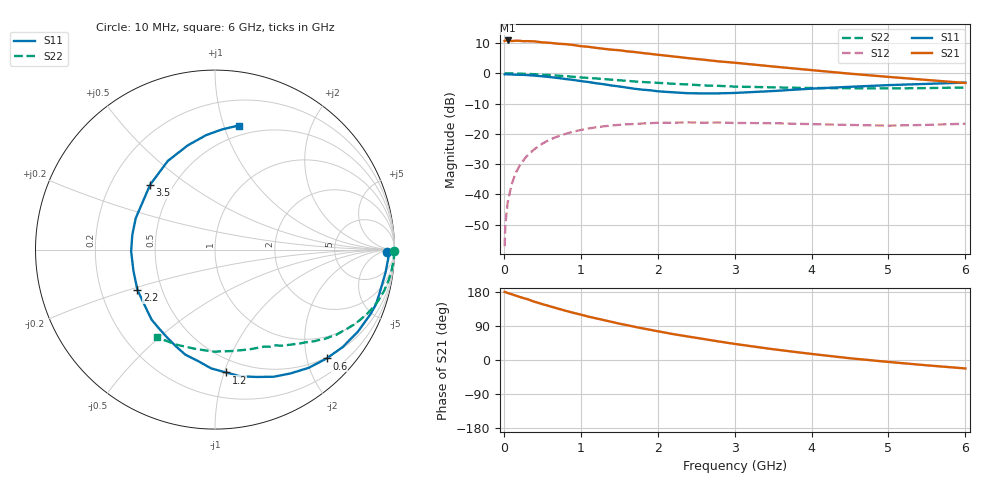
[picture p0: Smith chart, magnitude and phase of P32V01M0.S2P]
! SIEMENS Small Signal Semiconductors
! BFP181
! Si NPN RF Bipolar Junction Transistor in SOT143
! VCE = 2 V  IC = 1 mA
! Common Emitter S-Parameters:  March  1996
# GHz  S  MA  R  50
!  f  S11  S21  S12  S22
! GHz  MAG  ANG  MAG  ANG  MAG  ANG  MAG  ANG
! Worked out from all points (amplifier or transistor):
!   36 points, 10 MHz to 6 GHz, reference 50 ohm
!   highest |S21| = 10.9 dB at 50 MHz (marker M1)
!   |S21| within 3 dB of that: start of sweep to 1.385 GHz
!   unconditionally stable (mu >= 1): 3.02 GHz to end of sweep
!   at 250 MHz: K = 0.09, MSG = 19.7 dB, |S12| = -28.9 dB
!   at 1.4 GHz: K = 0.50, MSG = 12.5 dB, |S12| = -17.2 dB
!   at 6 GHz: K = 1.29, MAG = 3.5 dB, |S12| = -16.6 dB
!   lowest NFmin = 1.30 dB at 450 MHz
!   S11 on the Smith chart (normalised r, x): 10 MHz: 43, -15; 600 MHz: 0.48, -2.37; 1.2 GHz: 0.39, -1.01; 2.2 GHz: 0.36, -0.21; 3.5 GHz: 0.37, +0.36; 6 GHz: 0.41, +1.12
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0.01  0.9595 -0.8  3.44 179.7  0.0014 74.7  0.998 -0.3
0.02  0.9697 -1.5  3.486 179.3  0.0032 81.3  0.9978 -0.7
0.05  0.9652 -3.5  3.498 176.8  0.0074 88.9  0.9968 -1.9
0.1  0.959 -7.5  3.42 173.6  0.0145 84.2  0.9995 -3.5
0.2  0.9483 -15.2  3.46 166.8  0.0291 80.1  0.9906 -7.1
0.4  0.918 -29.9  3.379 153.7  0.0564 70.6  0.9691 -13.9
0.6  0.8687 -44.3  3.192 141.7  0.0809 61.1  0.9377 -20.1
0.8  0.8078 -58.7  3.042 130.1  0.1 52.8  0.8993 -25.7
0.9  0.7803 -65.2  2.944 124.7  0.1088 48.5  0.8791 -28.4
1.1  0.7198 -78.7  2.748 114.4  0.1229 41.8  0.8405 -33.0
1.2  0.6874 -84.9  2.636 109.9  0.1289 38.2  0.8243 -35.3
1.5  0.6081 -105.8  2.412 96.0  0.1411 30.0  0.7684 -40.9
1.7  0.5569 -118.8  2.254 87.7  0.1461 25.1  0.7354 -44.4
2  0.5061 -138.9  2.032 75.9  0.1528 19.2  0.6979 -48.7
2.2  0.4868 -152.6  1.905 68.4  0.1535 15.5  0.6737 -51.9
2.8  0.4681 169.9  1.575 48.7  0.1543 7.1  0.6217 -60.5
3  0.4751 158.3  1.501 42.5  0.1519 4.8  0.605 -63.4
3.5  0.5112 135.0  1.299 28.4  0.1503 1.0  0.5878 -71.2
4  0.5597 118.0  1.132 16.0  0.1452 -1.7  0.573 -80.5
4.5  0.6003 104.6  0.989 4.6  0.1406 -3.3  0.5686 -90.7
5.5  0.6714 86.5  0.779 -14.1  0.1409 0.0  0.572 -112.2
6  0.7038 79.2  0.694 -22.3  0.1475 0.6  0.5852 -123.2
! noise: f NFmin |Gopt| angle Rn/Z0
0.45  1.3  0.7  18  0.5
0.9  1.4  0.6  39  0.52
1.8  1.85  0.4  81  0.47
